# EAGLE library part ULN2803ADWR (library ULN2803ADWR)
Darlington Transistor Array Source: Datasheet
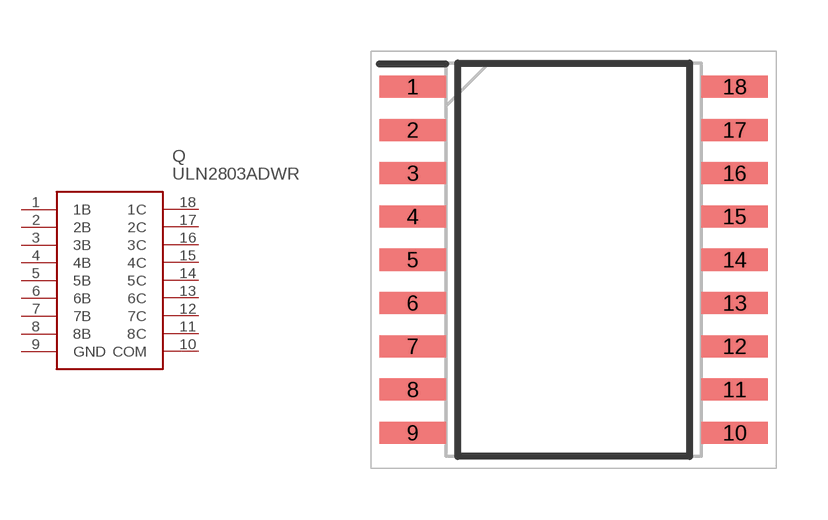
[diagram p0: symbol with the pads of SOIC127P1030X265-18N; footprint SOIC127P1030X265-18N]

Designator prefix Q

## ULN2803ADWR (Description: Darlington Transistor Array; Height: 2.65mm; Manufacturer_Name: Texas Instruments; Manufacturer_Part_Number: ULN2803ADWR; Mouser_Part_Number: 595-ULN2803ADWR; Mouser_Price-Stock: https://www.mouser.co.uk/ProductDetail/Texas-Instruments/ULN2803ADWR?qs=zqbRmZ%252BfZD8M77SqrzUfYg%3D%3D)  [SOIC127P1030X265-18N]
1  1B
2  2B
3  3B
4  4B
5  5B
6  6B
7  7B
8  8B
9  GND
10  COM
11  8C
12  7C
13  6C
14  5C
15  4C
16  3C
17  2C
18  1C

## Footprint SOIC127P1030X265-18N (pad centres in mm)
DW (R-PDSO-G18)
smd 1.95 x 0.65: 1 -4.725,5.08; 2 -4.725,3.81; 3 -4.725,2.54; 4 -4.725,1.27; 5 -4.725,0; 6 -4.725,-1.27; 7 -4.725,-2.54; 8 -4.725,-3.81; 9 -4.725,-5.08; 10 4.725,-5.08; 11 4.725,-3.81; 12 4.725,-2.54; 13 4.725,-1.27; 14 4.725,0; 15 4.725,1.27; 16 4.725,2.54; 17 4.725,3.81; 18 4.725,5.08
